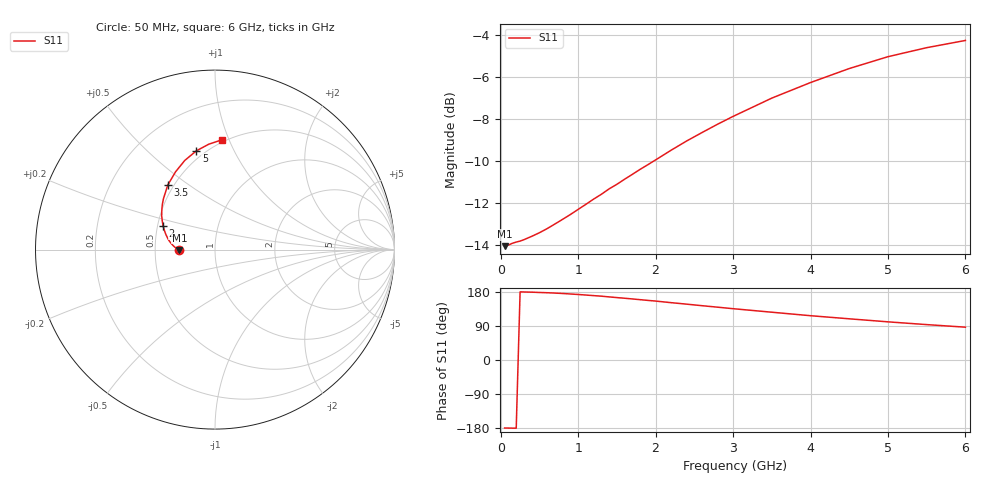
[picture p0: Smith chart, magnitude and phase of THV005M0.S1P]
! SIEMENS Discrete & RF Semiconductors
! BAS70
! Si Schottky Diode in SOT23
! IF = 5 mA
! S-Parameters:  February  1997
# GHz  S  MA  R  50
!  f  S11
! GHz  MAG  ANG
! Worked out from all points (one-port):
!   34 points, 50 MHz to 6 GHz, reference 50 ohm
!   lowest |S11| = -14.1 dB at 50 MHz (marker M1), VSWR 1.49, Z = 33.5 - j0.12 ohm
!   |S11| at or under -10 dB: start of sweep to 1.98 GHz
!   S11 on the Smith chart (normalised r, x): 50 MHz: 0.67, -0.00; 2 GHz: 0.54, +0.16; 3.5 GHz: 0.46, +0.42; 5 GHz: 0.45, +0.72; 6 GHz: 0.48, +0.94
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0.05  0.1981 -179.5
0.1  0.1993 -179.6
0.15  0.2012 -179.8
0.2  0.2026 -179.9
0.25  0.2037 179.8
0.3  0.2052 179.5
0.4  0.209 179.0
0.5  0.2132 178.2
0.6  0.2181 177.5
0.8  0.2295 175.5
1  0.2424 172.9
1.3  0.2633 168.4
1.4  0.2712 166.5
1.5  0.2781 164.7
1.6  0.286 163.0
1.8  0.3019 159.2
2  0.3179 155.5
2.2  0.3352 151.3
2.4  0.3526 147.4
2.6  0.3694 143.3
2.8  0.3866 139.4
3  0.4035 135.4
3.5  0.4461 126.1
4  0.4859 116.9
4.5  0.5246 108.7
5  0.5599 100.7
5.5  0.5882 93.4
6  0.612 86.6
